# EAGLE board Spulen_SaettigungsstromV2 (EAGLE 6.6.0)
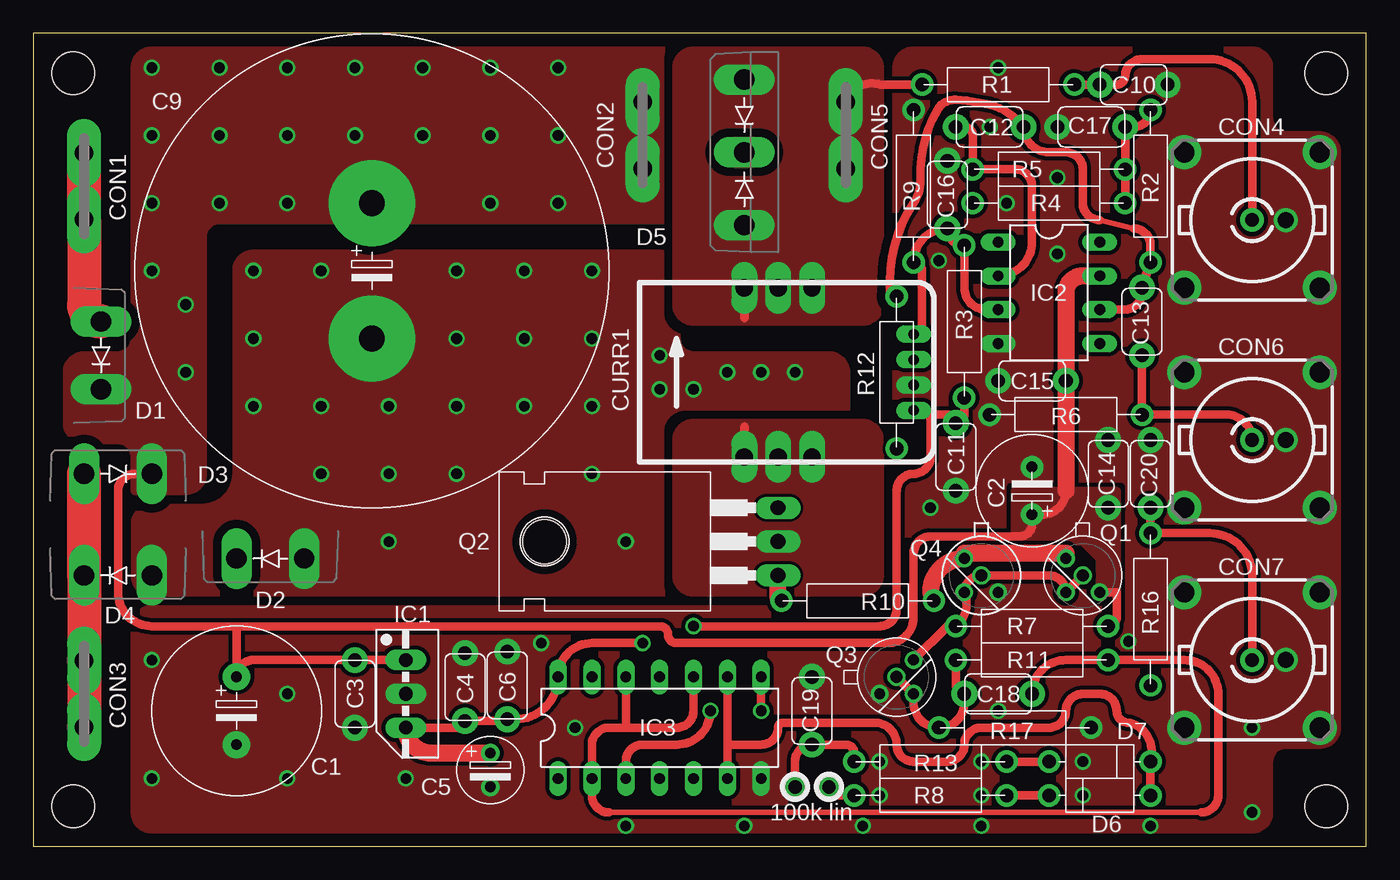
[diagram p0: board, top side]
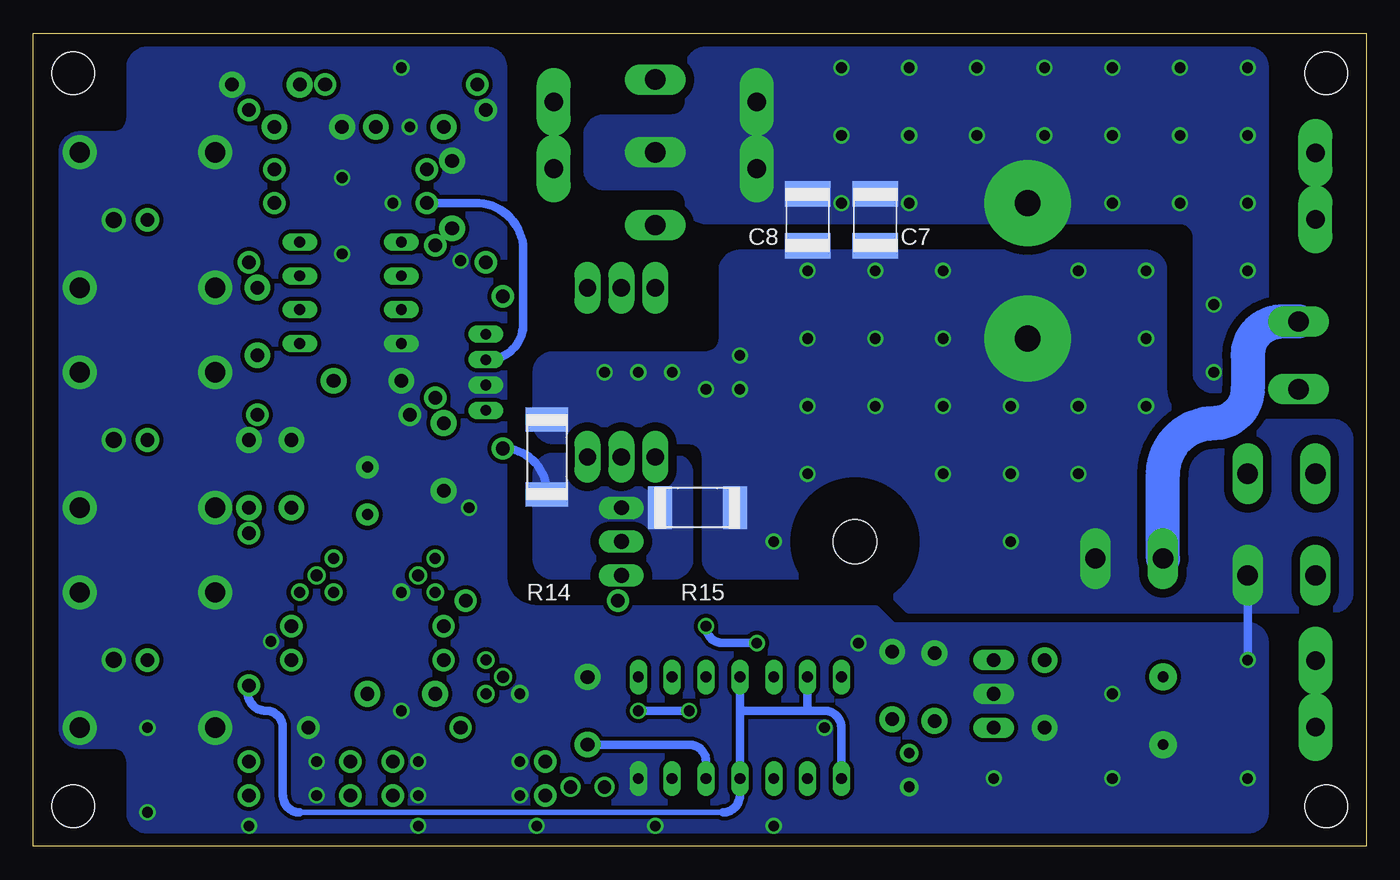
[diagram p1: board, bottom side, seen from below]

Size 100 x 61 mm. Coordinates in mm from the lower left corner, seen from the top.
Outline: 0,0 100,0 100,61 0,61 0,0
Copper layers (1*16): Top 0.035mm / dielectric 1.5mm / Bottom 0.035mm
Design rules "default *": minimum track width 10mil, minimum drill 24mil, track to track 8mil, track to pad 8mil, pad to pad 8mil, via to via 8mil, smd to smd 0mil, copper to edge 30mil, drill to drill 8mil, minimum pad ring 10mil, minimum via ring 8mil, stop-mask expansion 4mil, vias tented up to drill 0.8mm, thermal gap 10mil
Holes 3.2 mm at 3,58 3,3 97,3 97,58

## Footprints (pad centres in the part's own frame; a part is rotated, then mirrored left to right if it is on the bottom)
ES-5 = drill 0.813 pad 2.032: 1 -2.54,0; 2 2.54,0
ED-3,75 = drill 0.813 pad 1.676: 1 -1.778,0; 2 1.778,0
RM5.08(5X3) = drill 1.016 pad 1.93: 1 -2.54,0; 2 2.54,0
ES-2,5 = drill 0.813 pad 1.397: 1 -1.27,0; 2 1.27,0
1812 = smd 1.905 x 3.429: 1 -1.95,0; 2 1.95,0
ES-10-35MM = drill 1.93 pad 6.452: 1 -5.08,0; 2 5.08,0
F061.100 = drill 1.4 pad 2.54 long: A1 -2.5,0; A2 2.5,0
A1944 = drill 1.016 pad 1.778: 1 0,0 | drill 1.524 pad 2.54: 2 5.08,5.08; 3 -5.08,5.08; 4 -5.08,-5.08; 5 5.08,-5.08
CASR = drill 1.3 long: 1 5.08,-6.35; 2 2.54,-6.35; 3 0,-6.35; 8 0,6.35; 9 2.54,6.35; 10 5.08,6.35 | drill 0.8 long: 11 -7.62,-2.857; 12 -7.62,-0.953; 13 -7.62,0.953; 14 -7.62,2.857
DO220S = drill 1.524 long: A 2.54,-2.54; C -2.54,-2.54
SOT93S = drill 1.524 long: A1 -5.461,-2.54; A2 5.461,-2.54; C 0,-2.54
D-7.5 = drill 1.016 pad 1.676: 1 -3.81,0; 2 3.81,0
78MXXS = drill 1.016 long: GND 0,-2.54; IN -2.54,-2.54; OUT 2.54,-2.54
DIL08 = drill 0.813 long: 1 -3.81,-3.81; 2 -1.27,-3.81; 3 1.27,-3.81; 4 3.81,-3.81; 5 3.81,3.81; 6 1.27,3.81; 7 -1.27,3.81; 8 -3.81,3.81
DIL14 = drill 0.813 long: 1 -7.62,-3.81; 2 -5.08,-3.81; 3 -2.54,-3.81; 4 0,-3.81; 5 2.54,-3.81; 6 5.08,-3.81; 7 7.62,-3.81; 8 7.62,3.81; 9 5.08,3.81; 10 2.54,3.81; 11 0,3.81; 12 -2.54,3.81; 13 -5.08,3.81; 14 -7.62,3.81
TO18 = drill 0.813: 1 -1.27,-1.27; 2 1.27,-1.27; 3 1.27,1.27
TO220 = drill 1.118 long: 1 -2.54,-6.35; 2 0,-6.35; 3 2.54,-6.35 | hole 3.302: 0,11.176
R-12.5 = drill 1.016 pad 1.676: 1 -5.715,0; 2 5.715,0
2512 = smd 1.8 x 3.2: 1 -2.8,0; 2 2.8,0

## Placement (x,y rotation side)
C1  1000µ/25V  [ES-5]  15.24,10.16 270 top
C2  100µ/35V  [ED-3,75]  74.93,26.67 90 top
C3  100n  [RM5.08(5X3)]  24.13,11.43 90 top
C4  100n  [RM5.08(5X3)]  32.38,11.94 270 top
C5  100µ/16V  [ES-2,5]  34.29,5.71 270 top
C6  100n  [RM5.08(5X3)]  35.56,12.06 270 top
C7  100n  [1812]  36.83,46.99 270 bottom
C8  100n  [1812]  41.91,46.99 270 bottom
C9  18mF/35V  [ES-10-35MM]  25.4,43.18 270 top
C10  47p  [RM5.08(5X3)]  82.55,57.15 180 top
C11  100n  [RM5.08(5X3)]  69.22,29.21 90 top
C12  xxx  [RM5.08(5X3)]  71.75,53.98 180 top
C13  100n  [RM5.08(5X3)]  83.19,39.37 90 top
C14  100n  [RM5.08(5X3)]  80.64,27.94 270 top
C15  100n  [RM5.08(5X3)]  74.93,34.92 180 top
C16  10µ  [RM5.08(5X3)]  68.58,48.9 270 top
C17  xxx  [RM5.08(5X3)]  79.38,53.98 0 top
C18  3n3  [RM5.08(5X3)]  72.39,11.43 0 top
C19  3n3  [RM5.08(5X3)]  58.42,10.16 270 top
C20  47p  [RM5.08(5X3)]  83.82,27.94 270 top
CON1  [F061.100]  3.81,49.53 90 top
CON2  [F061.100]  45.72,53.34 90 top
CON3  [F061.100]  3.81,11.43 270 top
CON4  BNC  [A1944]  91.44,46.99 0 top
CON5  [F061.100]  60.96,53.34 90 top
CON6  BNC  [A1944]  91.44,30.48 0 top
CON7  BNC  [A1944]  91.44,13.97 0 top
CURR1  xxx  [CASR]  58.42,35.56 180 top
D1  STTH15AC06FP  [DO220S]  2.54,36.83 90 top
D2  STTH15AC06FP  [DO220S]  17.78,24.13 0 top
D3  STTH15AC06FP  [DO220S]  6.35,25.4 180 top
D4  STTH15AC06FP  [DO220S]  6.35,22.86 0 top
D5  VS-60APU02-N3  [SOT93S]  55.88,52.07 270 top
D6  BAT41  [D-7.5]  80.01,3.81 180 top
D7  BAT41  [D-7.5]  80.01,6.35 0 top
IC1  7805CT  [78MXXS]  30.48,11.43 270 top
IC2  TL071CP  [DIL08]  76.2,41.53 270 top
IC3  74HC14N  [DIL14]  46.99,8.89 0 top
Q1  2N2222  [TO18]  78.74,20.32 270 top
Q2  SUP60020E  [TO220]  49.53,22.86 90 top
Q3  2N2222  [TO18]  64.77,12.7 0 top
Q4  2N2907  [TO18]  71.12,20.32 270 top
R1  1k  [R-12.5]  72.39,57.15 0 top
R2  xxx  [R-12.5]  83.82,49.53 270 top
R3  180R  [R-12.5]  69.85,39.37 270 top
R4  1k  [R-12.5]  76.2,48.26 0 top
R5  xxx  [R-12.5]  76.2,50.8 180 top
R6  10k  [R-12.5]  77.47,32.38 0 top
R7  1k  [R-12.5]  74.93,16.51 0 top
R8  2k7  [R-12.5]  67.31,3.81 0 top
R9  1k  [R-12.5]  66.04,49.53 270 top
R10  22R  [R-12.5]  61.85,18.41 180 top
R11  1k  [R-12.5]  74.93,13.97 180 top
R12  n.b.  [R-12.5]  64.77,35.56 90 top
R13  10M  [R-12.5]  67.31,6.35 0 top
R14  0R  [2512]  61.47,29.21 270 bottom
R15  0R  [2512]  50.16,25.4 180 bottom
R16  1k  [R-12.5]  83.82,17.78 90 top
R17  1k  [R-12.5]  73.66,8.89 180 top

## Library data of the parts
C1-C20 D6 D7 R1-R17 = DISCRETE
CON1-CON3 CON5 = con-faston; OC_FARNELL: unknown; OC_NEWARK: unknown
CON4 CON6 CON7 = con-coax; OC_FARNELL: unknown; OC_NEWARK: unknown
CURR1 = Spulen_SaettigungsstromV2
D1-D5 = diode
IC1 = v-reg
IC2 = analog-devices; MPN: AD8031BNZ; OC_FARNELL: 1438575; OC_NEWARK: 15P0920
IC3 = 74xx-eu
Q1 Q3 = transistor-npn
Q2 = transistor-fet
Q4 = transistor-pnp

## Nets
+5V: C4.2 C5.1 C6.2 C11.2 CURR1.14 IC1.OUT IC3.14 R3.2
CURR: CURR1.12 R4.1
CURR+: CON5.A1 CON5.A2 CURR1.1 CURR1.2 CURR1.3 D5.A1 D5.A2 R1.1
CURR-: CURR1.8 CURR1.9 CURR1.10 Q2.2
GND: C1.2 C2.2 C3.1 C4.1 C5.2 C6.1 C7.2 C8.2 C9.2 C10.1 C11.1 C14.1 C15.2 C16.1 C17.1 C19.1 C20.1 CON4.2 CON4.3 CON4.4 CON4.5 CON6.2 CON6.3 CON6.4 CON6.5 CON7.2 CON7.3 CON7.4 CON7.5 CURR1.13 D2.A D4.A IC1.GND IC2.4 IC3.7 Q3.1 Q4.3 R6.1 R9.1 R14.1 R15.1 R17.1
N$1: C10.2 CON4.1 R1.2
N$2: C13.1 CON6.1 R6.2
N$3: C18.2 IC3.2 IC3.10 IC3.12 R11.1
N$4: Q2.3 R12.1 R14.2 R15.2
N$6: IC3.3 IC3.8
N$7: D7.1 R13.2
N$8: CON1.A1 CON1.A2 D1.A D2.C
N$9: C19.2 IC3.5 R13.1
N$10: R8.1
N$11: D6.1 D7.2 IC3.6 IC3.9
N$12: C20.2 CON7.1 R16.2
N$13: Q1.1 Q4.1 R10.1
N$14: C12.2 IC2.2 R5.2
N$15: CON3.A1 CON3.A2 D3.A D4.C
N$16: C12.1 C13.2 IC2.6 R2.2 R12.2
N$17: D6.2 R8.2
N$18: IC3.1 IC3.4 IC3.11 IC3.13 R16.1
N$19: C17.2 R2.1 R4.2 R5.1
N$22: C18.1 Q3.2 R11.2 R17.2
N$23: Q1.2 Q3.3 Q4.2 R7.1
N$27: Q2.1 R10.2
REF: C16.2 CURR1.11 IC2.3 R3.1 R9.2
VCC: C1.1 C2.1 C3.2 C7.1 C8.1 C9.1 C14.2 C15.1 CON2.A1 CON2.A2 D1.C D3.C D5.C IC1.IN IC2.7 Q1.3 R7.2

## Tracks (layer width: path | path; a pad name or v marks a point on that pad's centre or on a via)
+5V  (via drill 0.8)
  Top 0.635: v49.53,16.51 63.5,16.51 arc90 64.77,17.78 64.77,26.67 arc-90 66.04,27.94 arc90 67.31,29.21 67.31,32.38 | v45.72,15.24 41.91,15.24 arc90 IC3.14 arc-90 36.2,9.53 C6.2 arc-90 35.43,9.4 C4.2 arc-90 31.88,8.89 IC1.OUT | R3.2 69.85,32.38 arc-90 C11.2 arc90 68.58,32.38 67.31,32.38 | 67.31,32.38 66.04,32.38 CURR1.14
  Top 1.27: C5.1 29.84,6.99 arc-90 IC1.OUT
  Bottom 0.635: v45.72,15.24 48.26,15.24 arc90 v49.53,16.51
CURR
  Bottom 0.635: R4.1 66.55,48.26 arc90 63.25,44.45 63.25,39.05 arc90 CURR1.12
CURR+
  Top 0.635: CURR1.1 53.34,39.63 | R1.1 63.54,57.15 arc90 CON5.A2
  pour Top (isolate 0.635, no thermals): 49.53,59.69 62.23,59.69 arc-90 63.5,58.42 63.5,40.64 arc-90 62.23,39.37 49.53,39.37 arc-90 48.26,40.64 48.26,58.42 arc-90
CURR-
  Top 0.635: CURR1.10 53.34,31.49
  pour Top (no thermals): 49.53,31.75 62.23,31.75 arc-90 63.5,30.48 63.5,20.32 arc-90 62.23,19.05 49.53,19.05 arc-90 48.26,20.32 48.26,30.48 arc-90
GND  (via drill 0.8, 1.2)
  Bottom 0.635: D4.A v8.89,13.97
  other vias: 93.98,46.99 93.98,30.48 93.98,13.97 16.51,43.18 21.59,43.18 31.75,38.1 16.51,38.1 16.51,33.02 21.59,27.94 21.59,33.02 26.67,33.02 26.67,27.94 26.67,22.86 31.75,27.94 31.75,33.02 36.83,33.02 36.83,38.1 36.83,43.18 41.91,43.18 41.91,38.1 41.91,33.02 41.91,27.94 44.45,22.86 57.15,35.56 54.61,35.56 52.07,35.56 49.53,34.29 46.99,34.29 46.99,36.83 8.89,5.08 19.05,5.08 19.05,11.43 27.94,5.08 38.1,15.24 44.45,1.52 63.5,6.35 71.12,6.35 71.12,3.81 63.5,3.81 78.74,3.81 78.74,6.35 91.44,2.54 91.44,8.89 82.17,15.37 72.39,10.16 67.31,25.4 67.94,43.94 72.39,58.42 31.75,43.18 71.75,53.98 73.03,48.26 76.83,50.16 76.83,44.45 40.64,8.89 53.34,1.52 62.23,1.52 71.12,1.52 83.82,1.52
  pour Bottom (isolate 0.635, no thermals): 2.54,31.75 12.7,31.75 arc90 15.24,34.29 15.24,43.18 arc-90 16.51,44.45 46.99,44.45 arc-90 48.26,43.18 48.26,38.1 arc90 49.53,36.83 60.96,36.83 arc-90 62.23,35.56 62.23,31.75 arc-90 60.96,30.48 50.8,30.48 arc90 49.53,29.21 49.53,21.59 arc-90 48.26,20.32 36.83,20.32 34.29,17.78 2.54,17.78 arc-90 1.27,19.05 1.27,30.48 arc-90
  pour Bottom (isolate 0.305, no thermals): 66.04,59.69 91.44,59.69 arc-90 92.71,58.42 92.71,54.61 arc90 93.98,53.34 96.52,53.34 arc-90 97.79,52.07 97.79,8.89 arc-90 96.52,7.62 93.98,7.62 arc90 92.71,6.35 92.71,2.54 arc-90 91.44,1.27 8.89,1.27 arc-90 7.62,2.54 7.62,15.24 arc-90 8.89,16.51 35.56,16.51 36.83,17.78 62.23,17.78 arc90 64.77,20.32 64.77,58.42 arc-90
  pour Top (isolate 0.635, rank 2, no thermals): 8.89,25.4 12.7,25.4 arc90 15.24,27.94 15.24,43.18 arc-90 16.51,44.45 46.99,44.45 arc-90 48.26,43.18 48.26,38.1 arc90 49.53,36.83 59.69,36.83 arc-90 60.96,35.56 60.96,20.32 arc-90 59.69,19.05 8.89,19.05 arc-90 7.62,20.32 7.62,24.13 arc-90
  pour Top (isolate 0.305, rank 2, no thermals): 66.04,59.69 91.44,59.69 arc-90 92.71,58.42 92.71,54.61 arc90 93.98,53.34 96.52,53.34 arc-90 97.79,52.07 97.79,8.89 arc-90 96.52,7.62 93.98,7.62 arc90 92.71,6.35 92.71,2.54 arc-90 91.44,1.27 8.89,1.27 arc-90 7.62,2.54 7.62,16.51 arc-90 8.89,17.78 62.23,17.78 arc90 64.77,20.32 64.77,58.42 arc-90
N$1
  Top 0.635: R1.2 C10.2 81.28,57.15 arc90 81.92,57.78 arc-90 83.19,59.05 88.27,59.05 arc-90 91.44,55.88 CON4.1
N$2
  Top 0.635: CON6.1 arc90 89.53,32.38 R6.2 83.19,36.2 arc-90 C13.1
N$3
  Top 0.406: 43.18,2.54 87.63,2.54
  Top 0.635: 44.45,8.89 48.26,8.89 arc90 49.53,10.16 IC3.10 | 44.45,8.89 IC3.12 | 44.45,8.89 43.18,8.89 arc90 41.91,7.62 IC3.2 41.91,3.81 arc90 43.18,2.54 | 87.63,2.54 arc90 88.9,3.81 88.9,11.43 arc90 86.36,13.97 R11.1 77.47,13.97 arc90 C18.2
N$4
  Bottom 0.635: R12.1 arc90 61.47,26.54 R14.2
  pour Bottom (isolate 0.635, no thermals): 52.07,29.21 60.96,29.21 arc-90 62.23,27.94 62.23,21.59 arc-90 60.96,20.32 52.07,20.32 arc-90 50.8,21.59 50.8,27.94 arc-90
N$6  (via drill 0.8)
  Top 0.635: IC3.3 44.45,6.35 arc-90 45.72,7.62 48.26,7.62 arc90 v50.8,10.16 | v54.61,10.16 IC3.8
  Bottom 0.635: v50.8,10.16 v54.61,10.16
N$7
  Top 0.635: R13.2 D7.1
N$8
  Top 2.54: CON1.A2 CON1.A1 3.81,40.64 arc90 D1.A
  Bottom 2.54: D1.A 6.35,39.37 arc-90 8.89,36.83 8.89,34.29 arc90 11.43,31.75 arc-90 15.24,27.94 D2.C
N$9  (via drill 1)
  Top 0.635: R13.1 61.59,6.99 arc90 60.96,7.62 C19.2 arc90 57.15,6.35 v57.15,4.45
  Bottom 0.635: C19.2 50.8,7.62 arc90 49.53,6.35 IC3.5
N$10  (via drill 1)
  Top 0.635: R8.1 60.2,3.81 arc-90 v59.69,4.45
N$11
  Top 0.635: D6.1 D7.2 arc90 82.3,9.27 arc-98 81.28,10.16 arc90 80.01,11.43 78.74,11.43 arc90 77.47,10.16 arc-90 76.2,8.89 71.12,8.89 arc90 69.85,7.62 arc-90 68.58,6.35 66.04,6.35 arc-90 64.77,7.62 arc90 63.12,9.27 56.26,9.27 arc90 55.88,8.89 arc-90 54.61,7.62 52.07,7.62 | IC3.9 52.07,7.62 | 52.07,7.62 IC3.6
N$12
  Top 0.635: CON7.1 91.44,20.32 arc90 88.27,23.5 R16.2 C20.2
N$13
  Top 1.27: Q1.1 77.47,21.97 69.85,21.97 Q4.1 arc90 67.31,19.05 R10.1
N$14
  Top 0.635: C12.2 69.85,53.98 arc-90 70.48,53.34 R5.2 73.66,50.8 arc-90 74.93,49.53 74.93,45.34 arc-90 IC2.2
N$15
  Top 2.54: CON3.A2 CON3.A1 D4.C D3.A
N$16
  Top 0.406: 80.01,46.99 82.55,46.35
  Top 0.635: IC2.6 82.04,40.26 arc90 C13.2 R2.2 83.82,45.09 arc90 82.55,46.35 | 80.01,46.99 arc-90 78.74,48.26 78.74,50.8 arc90 77.47,52.07 76.2,52.07 arc-90 C12.1 arc39 71.75,55.63 arc10 69.22,56.01 arc64 67.82,55.24 arc31 66.55,50.04 arc-36 66.04,48.26 arc34 64.26,42.42 64.26,41.78 arc90 R12.2
N$17
  Top 0.635: R8.2 D6.2
N$18
  Bottom 0.406: 80.01,2.54 48.26,2.54
  Bottom 0.635: IC3.13 41.91,10.16 | 41.91,10.16 46.99,10.16 | 46.99,10.16 IC3.11 | 46.99,10.16 IC3.4 46.99,3.81 arc90 48.26,2.54 | IC3.1 39.37,8.89 arc-90 40.64,10.16 41.91,10.16 | 80.01,2.54 arc90 81.28,3.81 81.28,8.89 arc-90 82.55,10.16 arc113 R16.1
N$19
  Top 0.635: R4.2 R5.1 C17.2 82.55,53.98 arc90 R2.1
N$22  (via drill 0.9)
  Top 0.635: v64.77,12.7 Q3.2 66.04,10.79 arc90 R17.2 arc90 69.85,10.79 C18.1 arc-90 69.22,12.06 R11.2
N$23  (via drill 0.9)
  Top 0.635: Q3.3 68.58,16.51 arc-90 R7.1 arc74 Q4.2 arc-90 v71.12,20.32 76.2,20.32 arc-90 Q1.2 v78.74,20.32
N$27
  Top 1.27: R10.2 arc-90 55.88,18.67 Q2.1
REF
  Top 0.635: IC2.3 71.5,40.26 arc-90 69.85,41.91 R3.1 arc-90 C16.2 arc90 R9.2 arc-90 66.67,43.18 66.67,39.05 arc-90 CURR1.11
VCC  (via drill 0.8)
  Top 0.635: 15.24,16.51 46.99,16.51 arc-90 47.62,15.88 arc90 48.26,15.24 64.14,15.24 arc90 66.04,17.14 66.04,21.97 arc-90 67.31,23.24 73.91,23.24 arc90 74.93,24.13 C2.1 75.69,24.89 arc90 77.47,26.67 | IC1.IN C3.2 16.51,13.97 arc90 C1.1 15.24,16.51 | 15.24,16.51 8.89,16.51 arc-90 6.35,19.05 6.35,26.67 arc-90 7.62,27.94 D3.C | R7.2 arc90 81.28,17.14 81.28,19.05 Q1.3
  Top 1.27: IC2.7 78.74,42.8 arc90 77.47,41.53 C15.1 77.47,26.67
  other vias: 8.89,58.42 13.97,58.42 8.89,53.34 8.89,48.26 13.97,48.26 13.97,53.34 19.05,48.26 19.05,53.34 19.05,58.42 24.13,58.42 24.13,53.34 29.21,53.34 29.21,58.42 34.29,58.42 39.37,58.42 39.37,53.34 34.29,53.34 39.37,48.26 34.29,48.26 8.89,43.18 11.43,35.56 11.43,40.64
  pour Bottom (isolate 0.635, no thermals): 8.89,59.69 arc90 7.62,58.42 7.62,35.56 arc90 8.89,34.29 11.43,34.29 arc90 12.7,35.56 12.7,45.72 arc-90 13.97,46.99 49.53,46.99 arc90 50.8,48.26 arc-90 52.07,49.53 57.15,49.53 arc90 58.42,50.8 58.42,53.34 arc90 57.15,54.61 52.07,54.61 arc-90 50.8,55.88 50.8,58.42 arc90 49.53,59.69
  pour Top (isolate 0.635, rank 2, no thermals): 8.89,59.69 arc90 7.62,58.42 7.62,38.1 arc-90 6.35,36.83 3.81,36.83 arc90 2.54,35.56 2.54,31.75 arc90 3.81,30.48 6.35,30.48 arc-90 7.62,29.21 7.62,26.67 11.43,26.67 arc90 12.7,27.94 12.7,45.72 arc-90 13.97,46.99 49.53,46.99 arc90 50.8,48.26 arc-90 52.07,49.53 57.15,49.53 arc90 58.42,50.8 58.42,53.34 arc90 57.15,54.61 52.07,54.61 arc-90 50.8,55.88 50.8,58.42 arc90 49.53,59.69
  pour Top (isolate 0.305, no thermals): 73.66,22.86 78.74,22.86 80.01,21.59 80.01,19.05 81.28,19.05 81.28,26.67 74.93,26.67 73.66,26.67

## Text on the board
tNames: 100k lin
tStop: HKE | Coil Measure | V2.0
